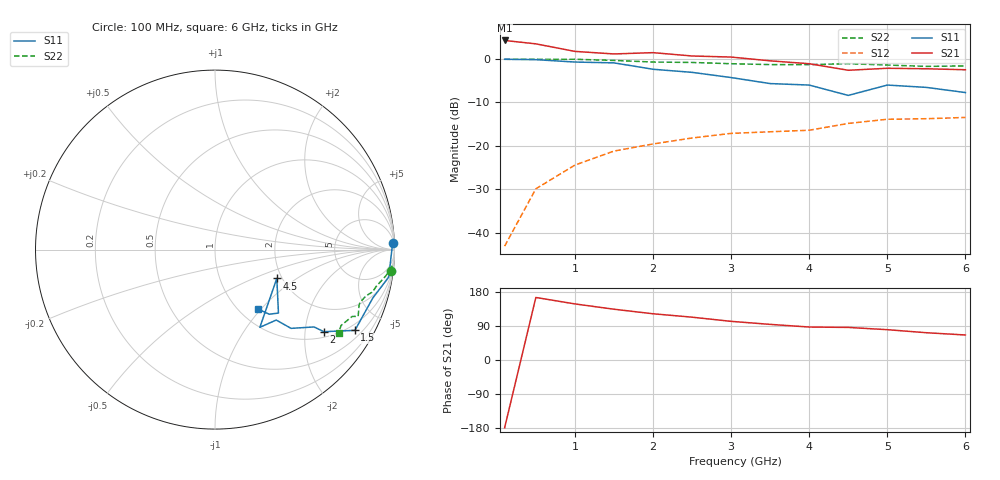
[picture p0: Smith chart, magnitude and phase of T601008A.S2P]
!AT-60100
!S-PARAMETERS at Vce=8V  Ic=0.5mA.  LAST UPDATED 07-21-92
# ghz s ma r 50
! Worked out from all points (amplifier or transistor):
!   13 points, 100 MHz to 6 GHz, reference 50 ohm
!   highest |S21| = 4.2 dB at 100 MHz (marker M1)
!   |S21| within 3 dB of that: start of sweep to 1.41 GHz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
!   unconditionally stable (mu >= 1): 3.278 GHz to end of sweep
!   at 1 GHz: K = 0.38, MSG = 13.1 dB, |S12| = -24.4 dB
!   at 3 GHz: K = 0.92, MSG = 8.8 dB, |S12| = -17.1 dB
!   at 6 GHz: K = 1.19, MAG = 2.8 dB, |S12| = -13.5 dB
!   S11 on the Smith chart (normalised r, x): 100 MHz: 15, +53; 1.5 GHz: 0.76, -3.58; 2 GHz: 1.16, -2.52; 4.5 GHz: 1.88, -0.70; 6 GHz: 1.21, -0.97
0.1  0.99 2.0  1.63 -179.0  0.007 88.0  0.99 -7.0
0.5  0.98 -9.0  1.49 165.0  0.032 86.0  0.99 -5.0
1  0.92 -17.0  1.22 148.0  0.06 78.0  0.99 -6.0
1.5  0.9 -30.0  1.14 134.0  0.087 70.0  0.96 -9.0
2  0.76 -37.0  1.18 122.0  0.105 67.0  0.92 -13.0
2.5  0.7 -38.0  1.08 113.0  0.123 66.0  0.91 -15.0
3  0.61 -46.0  1.05 102.0  0.139 63.0  0.88 -17.0
3.5  0.52 -49.0  0.95 94.0  0.145 61.0  0.86 -20.0
4  0.5 -60.0  0.88 87.0  0.151 62.0  0.86 -21.0
4.5  0.38 -25.0  0.74 86.0  0.181 70.0  0.88 -25.0
5  0.5 -45.0  0.78 80.0  0.202 62.0  0.85 -26.0
5.5  0.47 -50.0  0.77 72.0  0.205 57.0  0.82 -31.0
6  0.41 -54.0  0.75 66.0  0.212 55.0  0.83 -34.0
